PROGRAM P_MAIN_LowSpeed
VAR
	AODB		: ARRAY[0..1] OF ST_IEC870_5_101AODBEntry;(* Application object data base (only two data points) *)
	fbServer	: FB_IEC870_5_101Slave;(* IEC 60870-5-101 slave function block instance *)

	nCAA		: DWORD := 7; (* Common ASDU address of this (slave) station *)

	bSPI		AT%MX0.0 : BOOL;(* Single point information (data point used in monitoring direction slave->master) *)
	bSCS		AT%MX1.5 : BOOL;(* Single command state (data point used in control direction master->slave) *)

	fbTimer 	: TON := ( IN := TRUE, PT := T#1S );
	bInit		: BOOL 	:= TRUE;
	nInitErr	: UDINT;
END_VAR

IF bInit THEN
	bInit := FALSE;

	(* Configure protocol parameter *)
	fbServer.protPara.eLinkAddrSize := eIEC870_linkAddr_TwoOctets; (* Link address octet size *)
	fbServer.protPara.linkAddr 		:= 220; (* Link address *)
	fbServer.protPara.tMaxPollDelay := T#2S; (* Goes offline after max. delay time if polling requests are missing *)

	(* Configure system parameter *)
	fbServer.sysPara.asduAddr		 		:= nCAA;(* Configure own common ASDU address *)
	fbServer.sysPara.asduFmt.eCOTSize 		:= eIEC870_COT_TwoOctets;(* Cause of transfer octet size *)
	fbServer.sysPara.asduFmt.eAsduAddrSize 	:= eIEC870_AsduAddr_TwoOctets;(* Common ASDU address octet size *)
	fbServer.sysPara.asduFmt.eObjAddrSize 	:= eIEC870_ObjAddr_ThreeOctets;(* Information object address octet size *)
	fbServer.sysPara.dbgMode 				:= IEC870_DEBUGMODE_DEVSTATE(* OR IEC870_DEBUGMODE_LINKERROR OR IEC870_DEBUGMODE_ASDU OR IEC870_DEBUGMODE_LINKLAYER *);(* Enable output of device state change messages *)

	(* Configure one single point in monitoring direction *)
	nInitErr := F_iecInitAOEntry( 	M_SP_NA_1,(* Type is single point *)
									100,(* Information object address *)
									IEC870_GRP_INROGEN,(* Interrogation group *)
									0,(* Multiplier (not used) *)
									MAP_AREA_MEMORY,(* Map this single point value FROM PLC memory area (buffer) *)
									0,(* Map FROM byte offset *)
									0,(* Map FROM bit offset *)
									AODB[0] );(* Data base array element to initialize *)

	(* Configure one single command in control direction *)
	nInitErr := F_iecInitAOEntry( 	C_SC_NA_1,(* Type is single command *)
									10,(* Information object address *)
									0,(* Group (not used) *)
									0,(* Multiplier (not used) *)
									MAP_AREA_MEMORY, (* Map this single command value TO PLC memory area (buffer) *)
									1,(* Map TO byte offset *)
									5,(* Map TO bit offset *)
									AODB[1] );(* Data base array element to initialize *)

ELSE
	(* Execute IEC slave function block *)
	fbServer( 	pAOEntries 	:= ADR( AODB ),(* Start address of application object database *)
				cbAOEntries := SIZEOF( AODB ),(* Byte size of application object database *)
				pInputs 	:= 0,(* Not used *)
				cbInputs 	:= 0,(* Not used *)
				pOutputs 	:= 0,(* Not used *)
				cbOutputs 	:= 0,(* Not used *)
				pMemory 	:= ADR( %MB0 ),(* Start address of memory area (buffer). Memory buffer where the data point values are mapped to and from *)
				cbMemory 	:= 2,(* Byte size of memory area (buffer) = 2 byte (%MB0..%MB1) *)
				pData 		:= 0,(* Not used *)
				cbData 		:= 0,(* Not used *)
				hSerial 	:= P_SerialComm_HighSpeed.hSerial,(* Serial port connection/communication handle *)
				bEnable 	:= TRUE (* Enable communication *) );

	(* Check for device errors, remove them and log errror message to the TwinCAT->Error List CTRL+^, E *)
	REPEAT
		fbServer.system.device.errors.RemoveError();
		IF fbServer.system.device.errors.bOk  THEN
			ADSLOGSTR( 	ADSLOG_MSGTYPE_ERROR OR ADSLOG_MSGTYPE_LOG, 'IEC60870-5-101 slave error: 0x%s',
						DWORD_TO_HEXSTR( fbServer.system.device.errors.getError.nErrId, 8, FALSE) );
		END_IF
	UNTIL NOT fbServer.system.device.errors.bOk
	END_REPEAT

END_IF

fbTimer( IN := TRUE );
IF fbTimer.Q THEN
	fbTimer( IN := FALSE );
	
	bSPI := NOT bSPI;
	
END_IF

END_PROGRAM
